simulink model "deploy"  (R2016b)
settings: Solver=FixedStepAuto  StartTime=0.0  StopTime=inf  RelTol=1e-3  EnableMultiTasking=on
undefined symbols (not defined in the file or in its folder): analogpin, HYT221_add1, HYT221_add2, pin, serial
libraries: arduinolib x8, simulink x2, instrumentlib x1

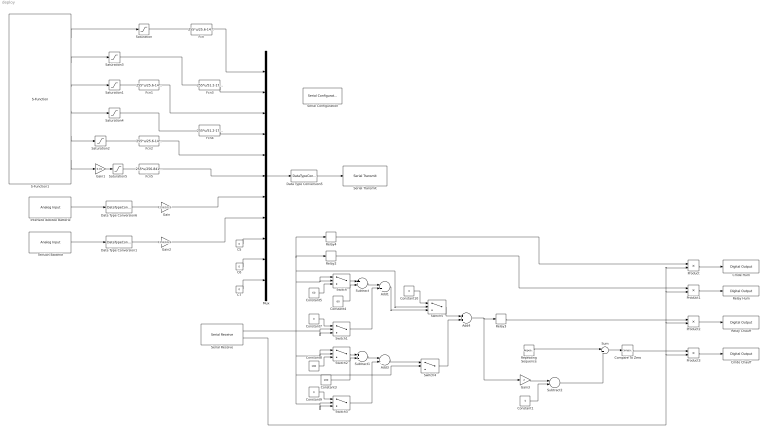
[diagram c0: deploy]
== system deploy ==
  Add1 : Sum
  Add3 : Sum
  Add4 : Sum
  C5 : Constant  Value=0
  C6 : Constant  Value=0
  C7 : Constant  Value=0
  Cmde Chauff : arduinolib/Digital Output  pinNumber=10  blockPlatform=arduino
  Cmde Hum : arduinolib/Digital Output  pinNumber=11  blockPlatform=arduino
  Compare To Zero : simulink/Logic and Bit Operations/Compare To Zero  relop=<=  OutDataTypeStr=boolean
  Constant1 : Constant  Value=5
  Constant10 : Constant  Value=0
  Constant3 : Constant  Value=180
  Constant4 : Constant  Value=60
  Constant5 : Constant  Value=60
  Constant7 : Constant  Value=0
  Constant8 : Constant  Value=180
  Constant9 : Constant  Value=0
  Data Type Conversion1 : DataTypeConversion  OutDataTypeStr=double
  Data Type Conversion5 : DataTypeConversion  OutDataTypeStr=uint8
  Data Type Conversion6 : DataTypeConversion  OutDataTypeStr=double
  Fcn : Fcn  Expr=255*u/25.6-143.4375
  Fcn1 : Fcn  Expr=255*u/25.6-143.4375
  Fcn2 : Fcn  Expr=255*u/25.6-143.4375
  Fcn3 : Fcn  Expr=255*u/51.2-174.3164
  Fcn4 : Fcn  Expr=255*u/51.2-174.3164
  Fcn5 : Fcn  Expr=255*u/256-841.7
  Gain : Gain  Gain=255/1023
  Gain1 : Gain  Gain=0.01
  Gain2 : Gain  Gain=255/1023
  Gain3 : Gain  Gain=2
  Intensité débitée Batterie : arduinolib/Analog Input  pinNumber=6  sampleTime=1  blockPlatform=arduino
  Mux : Mux  Inputs=11
  Product{,1..3} (4 alike) : Product
  Relay Chauff : arduinolib/Digital Output  pinNumber=13  blockPlatform=arduino
  Relay Hum : arduinolib/Digital Output  pinNumber=12  blockPlatform=arduino
  Relay2 : Relay  OnSwitchValue=60  OffSwitchValue=59
  Relay3 : Relay  OnSwitchValue=1  OffSwitchValue=0
  Relay4 : Relay  OnSwitchValue=180  OffSwitchValue=179
  Repeating Sequence : simulink/Sources/Repeating Sequence  rep_seq_t=[0 10]  rep_seq_y=[0 100]
  S-Function1 : S-Function  FunctionName=sfLect_Capteurs  Parameters=uint8(pin),uint8(analogpin),uint8(HYT221_add1),uint8(HYT221_add2)  SFunctionModules='sfLect_Capteurs_wrapper'  SFunctionDeploymentMode=off  EnableBusSupport=off
  Saturation : Saturate  UpperLimit=40  LowerLimit=14.4
  Saturation1 : Saturate  UpperLimit=40  LowerLimit=14.4
  Saturation2 : Saturate  UpperLimit=40  LowerLimit=14.4
  Saturation3 : Saturate  UpperLimit=86.2  LowerLimit=35
  Saturation4 : Saturate  UpperLimit=86.2  LowerLimit=35
  Saturation5 : Saturate  UpperLimit=1100  LowerLimit=845
  Serial Configuration : instrumentlib/Serial Configuration  Priority=-200000  ComPortMenu=<Please select a port...>  ComPort=COM8  ObjConstructor=serial('COM8');  BaudRate=9600  DataBits=8  Parity=none  StopBits=1  FlowControl=none  Timeout=10  ByteOrder=LittleEndian
  Serial Receive : arduinolib/Serial Receive  portNumber=0  showOutStatus=on  sampleTime=1  blockPlatform=arduino
  Serial Transmit : arduinolib/Serial Transmit  portNumber=0  blockPlatform=arduino
  Subtract : Sum  Inputs=+-
  Subtract1 : Sum  Inputs=+-
  Subtract2 : Sum  Inputs=+-
  Sum : Sum  Inputs=|+-
  Switch : Switch  Criteria=u2 > Threshold  Threshold=60
  Switch1 : Switch  Threshold=60
  Switch2 : Switch  Criteria=u2 > Threshold  Threshold=180
  Switch3 : Switch  Criteria=u2 > Threshold  Threshold=180
  Switch4 : Switch  Criteria=u2 > Threshold  Threshold=180
  Switch5 : Switch  Criteria=u2 > Threshold  Threshold=110
  Tension Batterie : arduinolib/Analog Input  pinNumber=0  sampleTime=1  blockPlatform=arduino
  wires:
  S-Function1/4 -> Saturation4/1
  S-Function1/5 -> Saturation2/1
  S-Function1/6 -> Gain1/1
  S-Function1/2 -> Saturation3/1
  S-Function1/3 -> Saturation1/1
  Data Type Conversion5/1 -> Serial Transmit/1
  Mux/1 -> Data Type Conversion5/1
  Gain1/1 -> Saturation5/1
  S-Function1/1 -> Saturation/1
  Fcn/1 -> Mux/1
  Fcn1/1 -> Mux/3
  Fcn2/1 -> Mux/5
  Fcn3/1 -> Mux/2
  Fcn4/1 -> Mux/4
  Fcn5/1 -> Mux/6
  Intensité débitée Batterie/1 -> Data Type Conversion6/1
  Tension Batterie/1 -> Data Type Conversion1/1
  Data Type Conversion6/1 -> Gain/1
  Data Type Conversion1/1 -> Gain2/1
  Saturation/1 -> Fcn/1
  Saturation1/1 -> Fcn1/1
  Saturation2/1 -> Fcn2/1
  Saturation3/1 -> Fcn3/1
  Saturation4/1 -> Fcn4/1
  Saturation5/1 -> Fcn5/1
  Gain/1 -> Mux/7
  Gain2/1 -> Mux/8
  C5/1 -> Mux/9
  C6/1 -> Mux/10
  C7/1 -> Mux/11
  Serial Receive/2 -> Product3/2, Product2/2, Product1/2, Product/2
  Compare To Zero/1 -> Product3/1
  Add4/1 -> Gain3/1, Relay3/1
  Relay2/1 -> Product1/1
  Relay3/1 -> Product2/1
  Switch/1 -> Subtract/1
  Subtract/1 -> Add1/1
  Constant4/1 -> Subtract/2
  Constant5/1 -> Switch/3
  Constant7/1 -> Switch1/1
  Switch1/1 -> Add1/2
  Switch2/1 -> Subtract1/1
  Subtract1/1 -> Add3/1
  Constant3/1 -> Subtract1/2
  Constant8/1 -> Switch2/3
  Constant9/1 -> Switch3/1
  Switch3/1 -> Add3/2
  Relay4/1 -> Product/1
  Add3/1 -> Switch4/1
  Add1/1 -> Switch5/3
  Serial Receive/1 -> Relay4/1, Relay2/1, Switch5/2, Switch/2, Switch/1, Switch1/2, Switch1/3, Switch2/1, Switch2/2, Switch4/2, Switch3/3, Switch3/2
  Switch5/1 -> Add4/1
  Switch4/1 -> Add4/2
  Constant10/1 -> Switch5/1
  Sum/1 -> Compare To Zero/1
  Repeating Sequence/1 -> Sum/1
  Subtract2/1 -> Sum/2
  Gain3/1 -> Subtract2/1
  Constant1/1 -> Subtract2/2
  Product1/1 -> Relay Hum/1
  Product/1 -> Cmde Hum/1
  Product2/1 -> Relay Chauff/1
  Product3/1 -> Cmde Chauff/1
